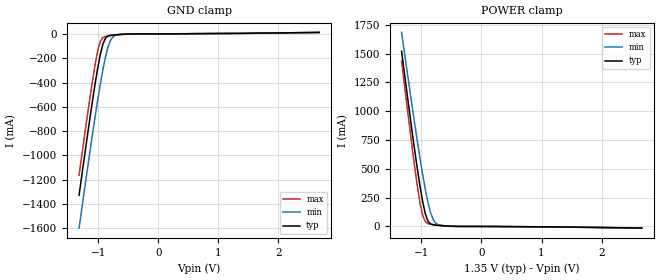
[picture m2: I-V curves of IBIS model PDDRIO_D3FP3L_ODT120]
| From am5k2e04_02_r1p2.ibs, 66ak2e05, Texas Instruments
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|   Model PDDRIO_D3FP3L_ODT120
[Model] PDDRIO_D3FP3L_ODT120
Model_type   Input
Polarity   Non-Inverting
Enable   Active-High
C_comp   3.284pF   3.217pF   3.375pF
C_comp_pullup   570.125fF   541.237fF   611.275fF
C_comp_pulldown 2.709pF   2.671pF   2.758pF
Vinh = 810.000mV
Vinl = 540.000mV
[Temperature Range]   25.000   125.000   -40.000
[Voltage Range]   1.350V   1.283V   1.450V
[GND Clamp Reference]   0.00V   0.00V   0.00V
|[C Comp Corner]
| variable   typ   min   max
|C_comp 3.284pF   3.375pF   3.217pF
|C_comp_pullup 570.125fF   611.275fF   541.237fF
|C_comp_pulldown 2.709pF   2.758pF   2.671pF
[POWER Clamp Reference]   1.350V   1.283V   1.450V
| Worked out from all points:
|   GND clamp passes 1 mA (typ) near -0.52 V on its own axis
|   POWER clamp passes 1 mA (typ) near -0.47 V on its own axis
[GND Clamp]
-1.318V   -1.327A    -1.598A    -1.163A
-1.142V   -709mA     -985.9mA   -542.4mA
-1.055V   -421.3mA   -693.5mA   -262.8mA
-1.011V   -289.9mA   -553.8mA   -145.7mA
-966.7mV  -174.3mA   -421mA     -63.6mA
-922.7mV  -85.4mA    -298.1mA   -29.42mA
-878.8mV  -35.01mA   -190.4mA   -20.83mA
-834.9mV  -16.59mA   -105.3mA   -17.41mA
-790.9mV  -10.91mA   -49.5mA    -14.73mA
-747mV    -8.321mA   -21.53mA   -12.2mA
-483.3mV  -432.1uA   -454.7uA   -931.7uA
2.68V     12.18mA    12.74mA    12.09mA
[Power Clamp]
-1.33V    1.521A     1.685A     1.435A
-1.155V   824.2mA    1.044A     688.4mA
-1.067V   498.8mA    737.5mA    347.8mA
-1.023V   348.9mA    591mA      202.4mA
-978.8mV  215.3mA    451.6mA    94.84mA
-934.9mV  109.4mA    322.7mA    41.2mA
-890.9mV  45.7mA     209.5mA    24.25mA
-847mV    21.07mA    119.4mA    19.23mA
-803mV    13.7mA     58.99mA    16.3mA
-759.1mV  10.7mA     26.88mA    13.74mA
-451.5mV  693.1uA    1.017mA    894uA
2.668V    -14.07mA   -14.85mA   -14.48mA
